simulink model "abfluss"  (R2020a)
settings: Solver=ode45  StartTime=0.0  StopTime=10.0  MaxStep=1  RelTol=1e-3  EnableMultiTasking=on

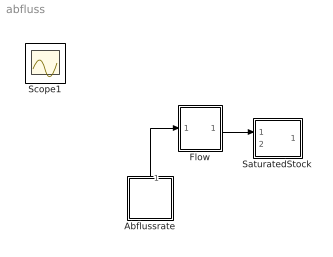
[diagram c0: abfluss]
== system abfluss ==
  Abflussrate : Subsystem  mask{k=0.5}
      mask prompts: k "Constant"
  Flow : Subsystem
  SaturatedStock : Subsystem  mask{m0=4, maxval=Inf, minval=0}
      mask prompts: m0 "Anfangswert"; maxval "obere Grenze"; minval "untere Grenze"
  Scope1 : Scope
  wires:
  Abflussrate/1(Out1) -> Flow/1(In1)
  Flow/1(Out1) -> SaturatedStock/1(In1)

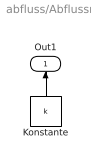
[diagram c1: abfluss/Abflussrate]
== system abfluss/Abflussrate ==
  Konstante : Constant  Value=k
  Out1 : Outport
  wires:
  Konstante/1 -> Out1/1

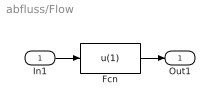
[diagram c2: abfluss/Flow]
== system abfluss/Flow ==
  In1 : Inport
  Fcn : Fcn  Expr=u(1)
  Out1 : Outport
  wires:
  In1/1 -> Fcn/1
  Fcn/1 -> Out1/1

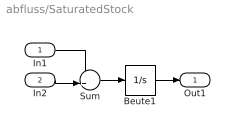
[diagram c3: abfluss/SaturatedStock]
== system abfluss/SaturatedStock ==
  In1 : Inport
  In2 : Inport  Port=2
  Beute1 : Integrator  InitialCondition=m0  LimitOutput=on  UpperSaturationLimit=maxval  LowerSaturationLimit=minval
  Sum : Sum  Inputs=-+|  SaturateOnIntegerOverflow=on
  Out1 : Outport
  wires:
  Sum/1 -> Beute1/1
  In1/1 -> Sum/1
  Beute1/1 -> Out1/1
  In2/1 -> Sum/2
